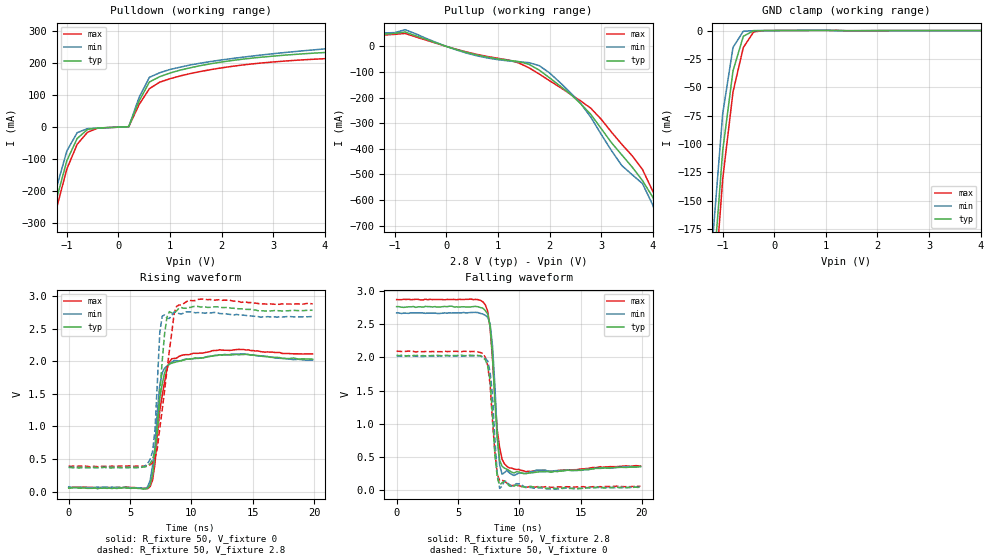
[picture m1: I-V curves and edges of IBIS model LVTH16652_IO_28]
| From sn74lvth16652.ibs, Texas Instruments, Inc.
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|  Model  LVTH16652 IO_28
[Model]   LVTH16652_IO_28
Model_type  I/O
Polarity   Non-Inverting
Enable   Active-Low
Vinl = 0.8V
Vinh = 2.0V
Vmeas = 1.5V
Cref = 50pF
Rref = 500
Vref = 0
| variable   typ   min   max
C_comp   10pf   NA   NA
[Temperature Range]   40   -25   100
| Ambient temperature   25   -40   85
[Voltage range]   2.8   2.7   2.9
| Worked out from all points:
|   slope of the pulldown table from 0 to 0.42 V, typ, clamps not added: 4.8 ohm
|   slope of the pullup table from 0 to 0.42 V, typ, clamps not added: 16.9 ohm
|   GND clamp passes 1 mA (typ) near -0.44 V on its own axis
|   rising waveform, R_fixture 50, V_fixture 0: 20-80 % time 653ps typ, 544ps min, 782ps max; typ from 0.052 V to 2.03 V
|   falling waveform, R_fixture 50, V_fixture 2.8: 20-80 % time 479ps typ, 409ps min, 579ps max; typ from 2.76 V to 0.358 V
|   rising waveform, R_fixture 50, V_fixture 2.8: 20-80 % time 575ps typ, 402ps min, 990ps max; typ from 0.37 V to 2.79 V
|   falling waveform, R_fixture 50, V_fixture 0: 20-80 % time 439ps typ, 429ps min, 517ps max; typ from 2.04 V to 0.042 V
[Pullup]
|   Voltage   I(typ)   I(min)   I(max)
-5V       68.55uA    66.79uA    67.33uA
-2.4V     58.24uA    55.2uA     58.55uA
-2.2V     52.25mA    54.89uA    49.25mA
-2V       48.28mA    52.88mA    45.68mA
-800mV    56.65mA    65.45mA    50.86mA
1.8V      -92.52mA   -74.97mA   -107.6mA
2.6V      -223mA     -221.5mA   -212.3mA
3V        -320.6mA   -342.8mA   -284.2mA
3.8V      -523.6mA   -535.4mA   -479.9mA
4.2V      -684.6mA   -733.9mA   -642.7mA
4.4V      -791.6mA   -852.7mA   -732.7mA
10V       -3.788A    -4.178A    -3.337A
[Pulldown]
|   Voltage   I(typ)   I(min)   I(max)
-5V       -3.748A    -4.01A     -3.373A
-1.4V     -373.4mA   -350.7mA   -401.7mA
-1.2V     -224.6mA   -188.8mA   -253.5mA
-1V       -104.5mA   -74.3mA    -130.5mA
-800mV    -35.47mA   -17.33mA   -53.65mA
-400mV    -2.631mA   -3.026mA   -3.177mA
200mV     1.341mA    1.503mA    1.221mA
600mV     140.8mA    155.4mA    120mA
1V        168.8mA    179.9mA    151mA
6.4V      261.8mA    314.4mA    231.7mA
8V        315.5mA    380.6mA    265.2mA
10V       385.9mA    441.4mA    310.8mA
[GND Clamp]
|   Voltage   I(typ)   I(min)   I(max)
-5V       -3.669A    -3.982A    -3.353A
-1.2V     -226.1mA   -187.6mA   -253mA
-1V       -106mA     -73.43mA   -131.1mA
-800mV    -35.52mA   -14.9mA    -54.18mA
-600mV    -5.092mA   -610.2uA   -14.94mA
-400mV    -130uA     -106uA     -1.208mA
-200mV    -43.46uA   -51.89uA   -43.91uA
5V        52.59nA    38.63nA    111.3nA
[Ramp]
| variable   typ   min   max
dV/dt_r   1.260E+00/6.900E-10  1.212E+00/5.390E-10  1.302E+00/8.320E-10
dV/dt_f   1.470E+00/4.610E-10  1.450E+00/4.110E-10  1.590E+00/6.030E-10
R_load = 50
[Rising Waveform]
R_fixture = 50
V_fixture = 0
V_fixture_min = 0
V_fixture_max = 0
C_fixture = 0
L_fixture = 0
|   Time   V(typ)   V(min)   V(max)
0s        51.73mV    71.87mV    61.95mV
6.25ns    39.83mV    45.47mV    50.97mV
6.641ns   109.3mV    173.6mV    77.52mV
6.836ns   258.9mV    400.5mV    178.5mV
7.031ns   568.9mV    693.2mV    426.3mV
7.422ns   1.44V      1.633V     1.245V
7.813ns   1.818V     1.894V     1.683V
8.398ns   1.973V     1.987V     2.041V
14.06ns   2.105V     2.116V     2.182V
19.88ns   2.034V     2.019V     2.114V
[Falling Waveform]
R_fixture = 50
V_fixture = 2.8
V_fixture_min = 2.7
V_fixture_max = 2.9
C_fixture = 0
L_fixture = 0
|   Time   V(typ)   V(min)   V(max)
0s        2.764V     2.67V      2.87V
6.641ns   2.762V     2.674V     2.869V
7.422ns   2.654V     2.603V     2.695V
7.617ns   2.477V     2.506V     2.45V
7.813ns   2.04V      2.177V     1.983V
8.203ns   779.4mV    822.5mV    903.5mV
8.398ns   455.9mV    379.3mV    645.5mV
8.594ns   363.3mV    243.7mV    469.1mV
10.55ns   255.4mV    253.6mV    281.4mV
19.88ns   358.1mV    359.4mV    366.7mV
[Rising Waveform]
R_fixture = 50
V_fixture = 2.8
V_fixture_min = 2.7
V_fixture_max = 2.9
C_fixture = 0
L_fixture = 0
|   Time   V(typ)   V(min)   V(max)
0s        370mV      373.8mV    390.3mV
6.445ns   398.1mV    432.9mV    400.2mV
6.836ns   492mV      613.6mV    443.9mV
7.031ns   617.8mV    949.6mV    504.6mV
7.422ns   1.49V      2.44V      968.8mV
7.617ns   1.998V     2.693V     1.251V
8.008ns   2.679V     2.662V     1.858V
8.594ns   2.745V     2.759V     2.732V
8.789ns   2.775V     2.758V     2.843V
19.88ns   2.785V     2.689V     2.883V
[Falling Waveform]
R_fixture = 50
V_fixture = 0
V_fixture_min = 0
V_fixture_max = 0
C_fixture = 0
L_fixture = 0
|   Time   V(typ)   V(min)   V(max)
0s        2.036V     2.022V     2.093V
6.445ns   2.033V     2.028V     2.089V
7.422ns   1.873V     1.946V     1.882V
7.617ns   1.659V     1.782V     1.597V
7.813ns   1.136V     1.434V     1.048V
8.008ns   539.7mV    775.5mV    580.6mV
8.203ns   197.5mV    255.4mV    242.2mV
8.398ns   79.8mV     30.67mV    146.8mV
8.789ns   139.2mV    143.3mV    140.2mV
19.88ns   41.66mV    47mV       62.71mV
